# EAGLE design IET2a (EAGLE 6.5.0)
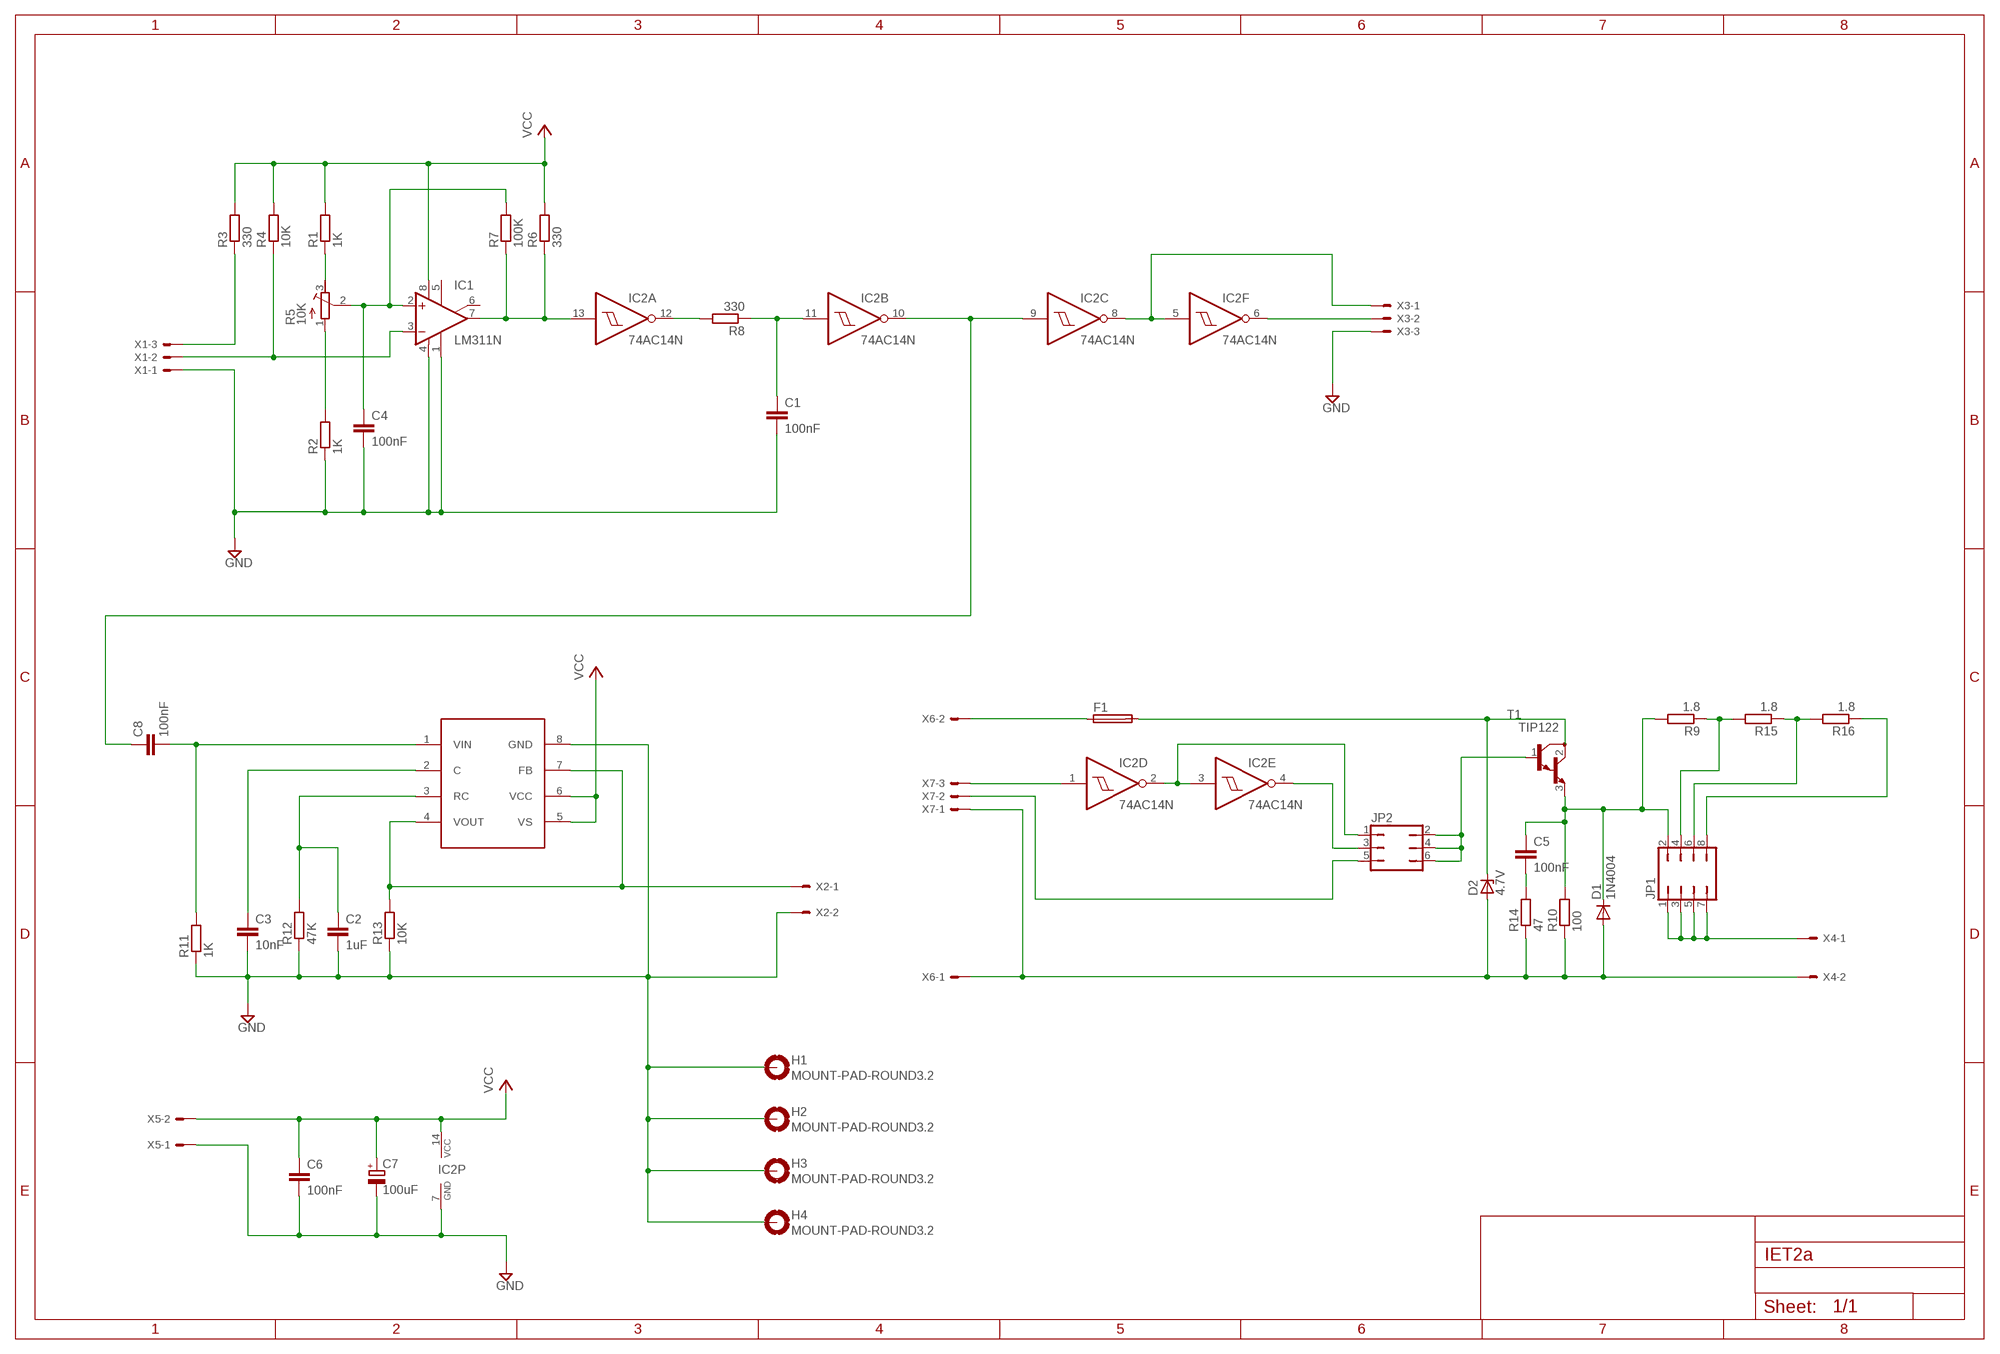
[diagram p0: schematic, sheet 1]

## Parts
C1  100nF  C-EU050-045X075  [C050-045X075]
C2  1uF  C-EU050-045X075  [C050-045X075]
C3  10nF  C-EU050-045X075  [C050-045X075]
C4  100nF  C-EU050-045X075  [C050-045X075]
C5  100nF  C-EU050-045X075  [C050-045X075]
C6  100nF  C-EU050-045X075  [C050-045X075]
C7  100uF  CPOL-EUE10-22.5  [EB22,5D]
C8  100nF  C-EU050-045X075  [C050-045X075]
D1  1N4004  [DO41-10]
D2  4.7V  1N4728  [DO41Z10]
F1  TE5  [TE5]
H1  MOUNT-PAD-ROUND3.2  [3,2-PAD]
H2  MOUNT-PAD-ROUND3.2  [3,2-PAD]
H3  MOUNT-PAD-ROUND3.2  [3,2-PAD]
H4  MOUNT-PAD-ROUND3.2  [3,2-PAD]
IC1  LM311N  [DIL08]
IC2  74AC14N  [DIL14]
IC4  LM2917A  [DIL08]
JP1  JP4Q  [JP4Q]
JP2  JP3Q  [JP3Q]
R1  1K  R-EU_0613/15  [P0613/15]
R2  1K  R-EU_0613/15  [P0613/15]
R3  330  R-EU_0613/15  [P0613/15]
R4  10K  R-EU_0613/15  [P0613/15]
R5  10K  R-TRIMM3299W  [RTRIM3299W]
R6  330  R-EU_0613/15  [P0613/15]
R7  100K  R-EU_0613/15  [P0613/15]
R8  330  R-EU_0613/15  [P0613/15]
R9  1.8  R-EU_0613/15  [P0613/15]
R10  100  R-EU_VTA56  [VTA56]
R11  1K  R-EU_0613/15  [P0613/15]
R12  47K  R-EU_0613/15  [P0613/15]
R13  10K  R-EU_0613/15  [P0613/15]
R14  47  R-EU_VTA56  [VTA56]
R15  1.8  R-EU_0613/15  [P0613/15]
R16  1.8  R-EU_0613/15  [P0613/15]
T1  TIP122  [TO220]
X1  KK-156-3  [KK-156-3]
X2  KK-156-2  [KK-156-2]
X3  KK-156-3  [KK-156-3]
X4  KK-156-2  [KK-156-2]
X5  KK-156-2  [KK-156-2]
X6  KK-156-2  [KK-156-2]
X7  KK-156-3  [KK-156-3]

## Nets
GND: C1.2 C2.2 C3.2 C4.2 C6.2 C7.- H1.B3,2(MOUNT) H2.B3,2(MOUNT) H3.B3,2(MOUNT) H4.B3,2(MOUNT) IC1.1(GND) IC1.4(V-) IC2.7(P:GND) IC4.8(GND) R2.1 R11.1 R12.1 R13.1 X1.1 X2.2 X3.3 X5.1
N$1: IC1.7(OUT) IC2.13(A:I) R6.1 R7.1
N$2: IC2.2(D:O) IC2.3(E:I) JP2.1
N$3: R3.1 X1.3
N$4: C5.2 R14.2
N$5: C1.1 IC2.11(B:I) R8.1
N$6: IC2.12(A:O) R8.2
N$7: R1.1 R5.3(A)
N$8: C4.1 IC1.2(+IN) R5.2(S) R7.2
N$9: IC1.3(-IN) R4.1 X1.2
N$10: R2.2 R5.1(E)
N$11: F1.1 X6.2
N$12: D2.C F1.2 T1.2(C)
N$13: D1.A D2.A R10.1 R14.1 X4.2 X6.1 X7.1
N$14: C5.1 D1.C JP1.2 R9.2 R10.2 T1.3(E)
N$15: JP1.4 R9.1 R15.2
N$16: IC2.1(D:I) X7.3
N$17: C8.1 IC2.9(C:I) IC2.10(B:O)
N$18: C3.1 IC4.2(C)
N$19: JP2.2 JP2.4 JP2.6 T1.1(B)
N$20: IC2.4(E:O) JP2.3
N$21: JP2.5 X7.2
N$22: C2.1 IC4.3(RC) R12.2
N$23: C8.2 IC4.1(VIN) R11.2
N$24: JP1.6 R15.1 R16.2
N$25: IC4.4(VOUT) IC4.7(FB) R13.2 X2.1
N$26: JP1.8 R16.1
N$27: JP1.1 JP1.3 JP1.5 JP1.7 X4.1
N$28: IC2.5(F:I) IC2.8(C:O) X3.1
N$29: IC2.6(F:O) X3.2
VCC: C6.1 C7.+ IC1.8(V+) IC2.14(P:VCC) IC4.5(VS) IC4.6(VCC) R1.2 R3.2 R4.2 R6.2 X5.2
Unconnected: IC1.5(ON) IC1.6(ON/STR)

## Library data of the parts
C1-C6 C8 = resistor:C-EU: CAPACITOR, European symbol
C7 = resistor:CPOL-EU: POLARIZED CAPACITOR, European symbol
D1 = diode:1N4004: DIODE
D2 = diode:1N4728: Z DIODE
F1 = fuse:TE5: FUSE; OC_FARNELL: unknown; OC_NEWARK: unknown
H1-H4 = holes:MOUNT-PAD-ROUND: MOUNTING PAD, round
IC1 = linear:LM311: COMPARATOR
IC2 = 74xx-eu:74*14: Hex schmitt trigger INVERTER
IC4 = IET:LM2917A
JP1 = jumper:JP4Q: JUMPER
JP2 = jumper:JP3Q: JUMPER
R1-R4 R6-R9 R11-R13 R15 R16 = resistor:R-EU_: RESISTOR, European symbol
R5 = resistor:R-TRIMM: Trimm resistor
R10 R14 = rcl:R-EU_: RESISTOR, European symbol
T1 = transistor:TIP122: NPN BIPOLAR DARLINGTON TRANSISTOR
X1 X3 X7 = con-molex:KK-156-3: KK 156 HEADER Source: http://www.molex.com/pdm_docs/sd/026604100_sd.pdf; OC_FARNELL: unknown; OC_NEWARK: unknown
X2 X4-X6 = con-molex:KK-156-2: KK 156 HEADER; OC_FARNELL: unknown; OC_NEWARK: unknown

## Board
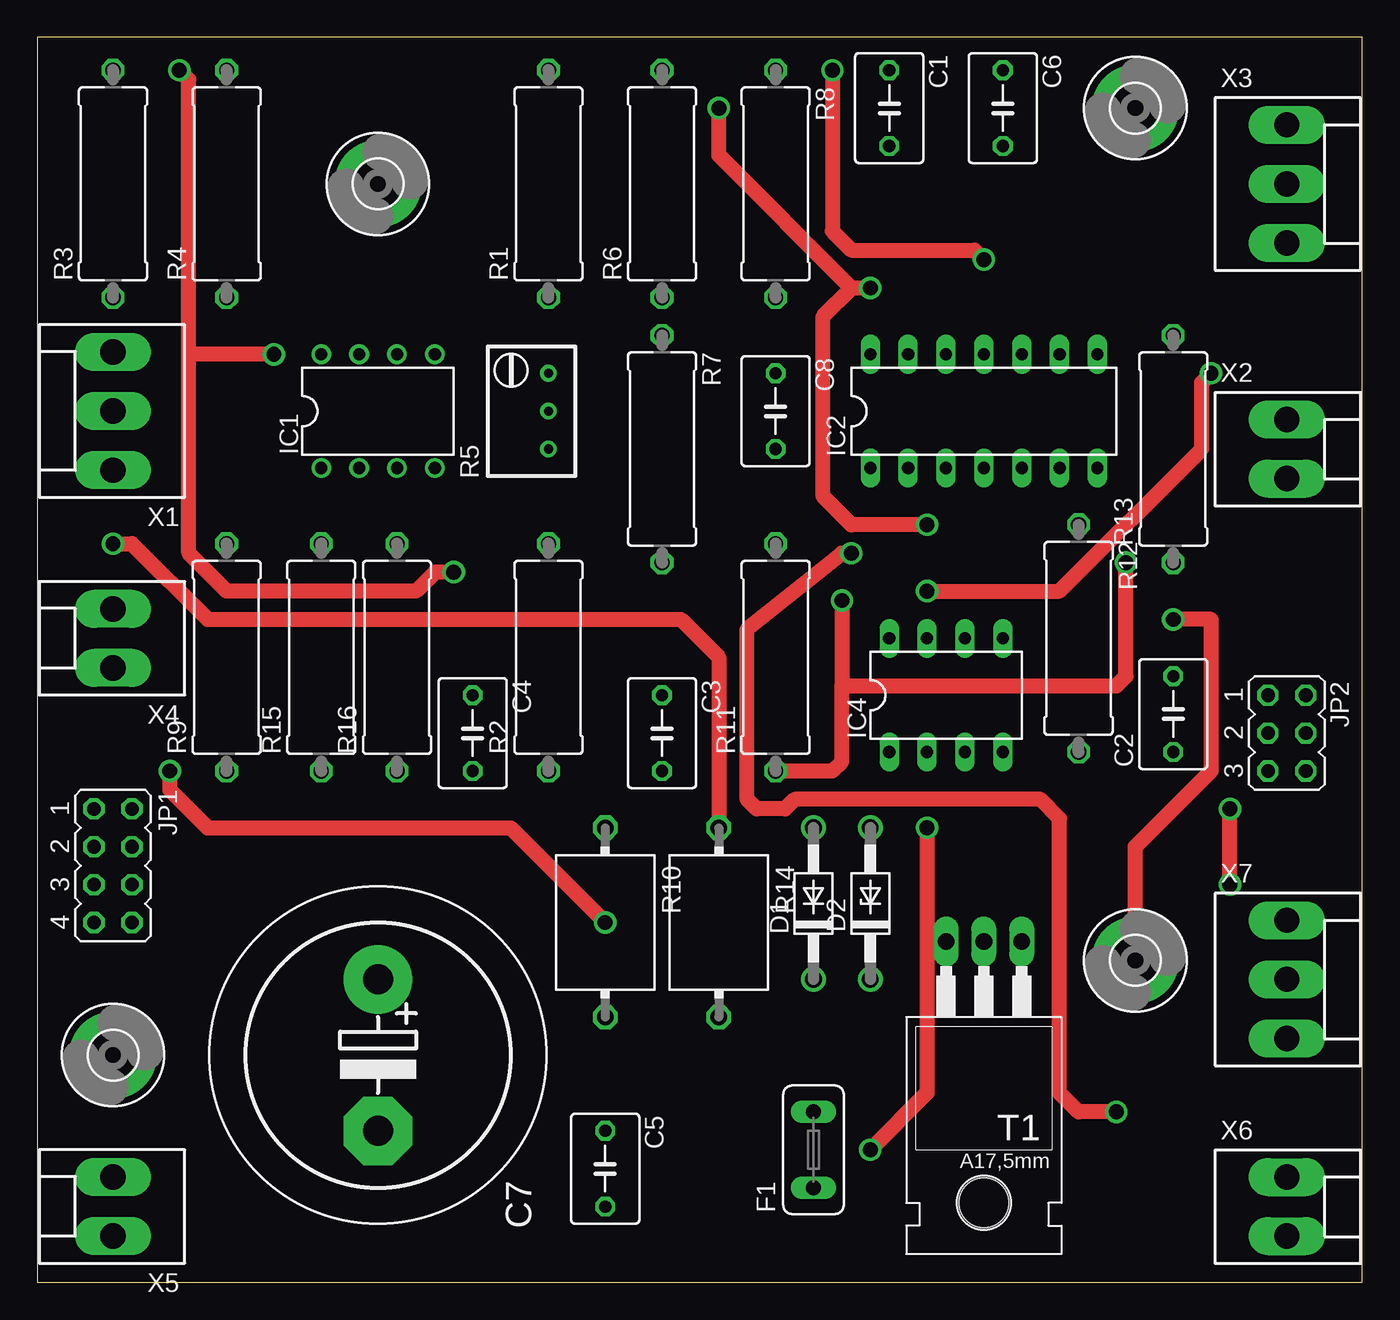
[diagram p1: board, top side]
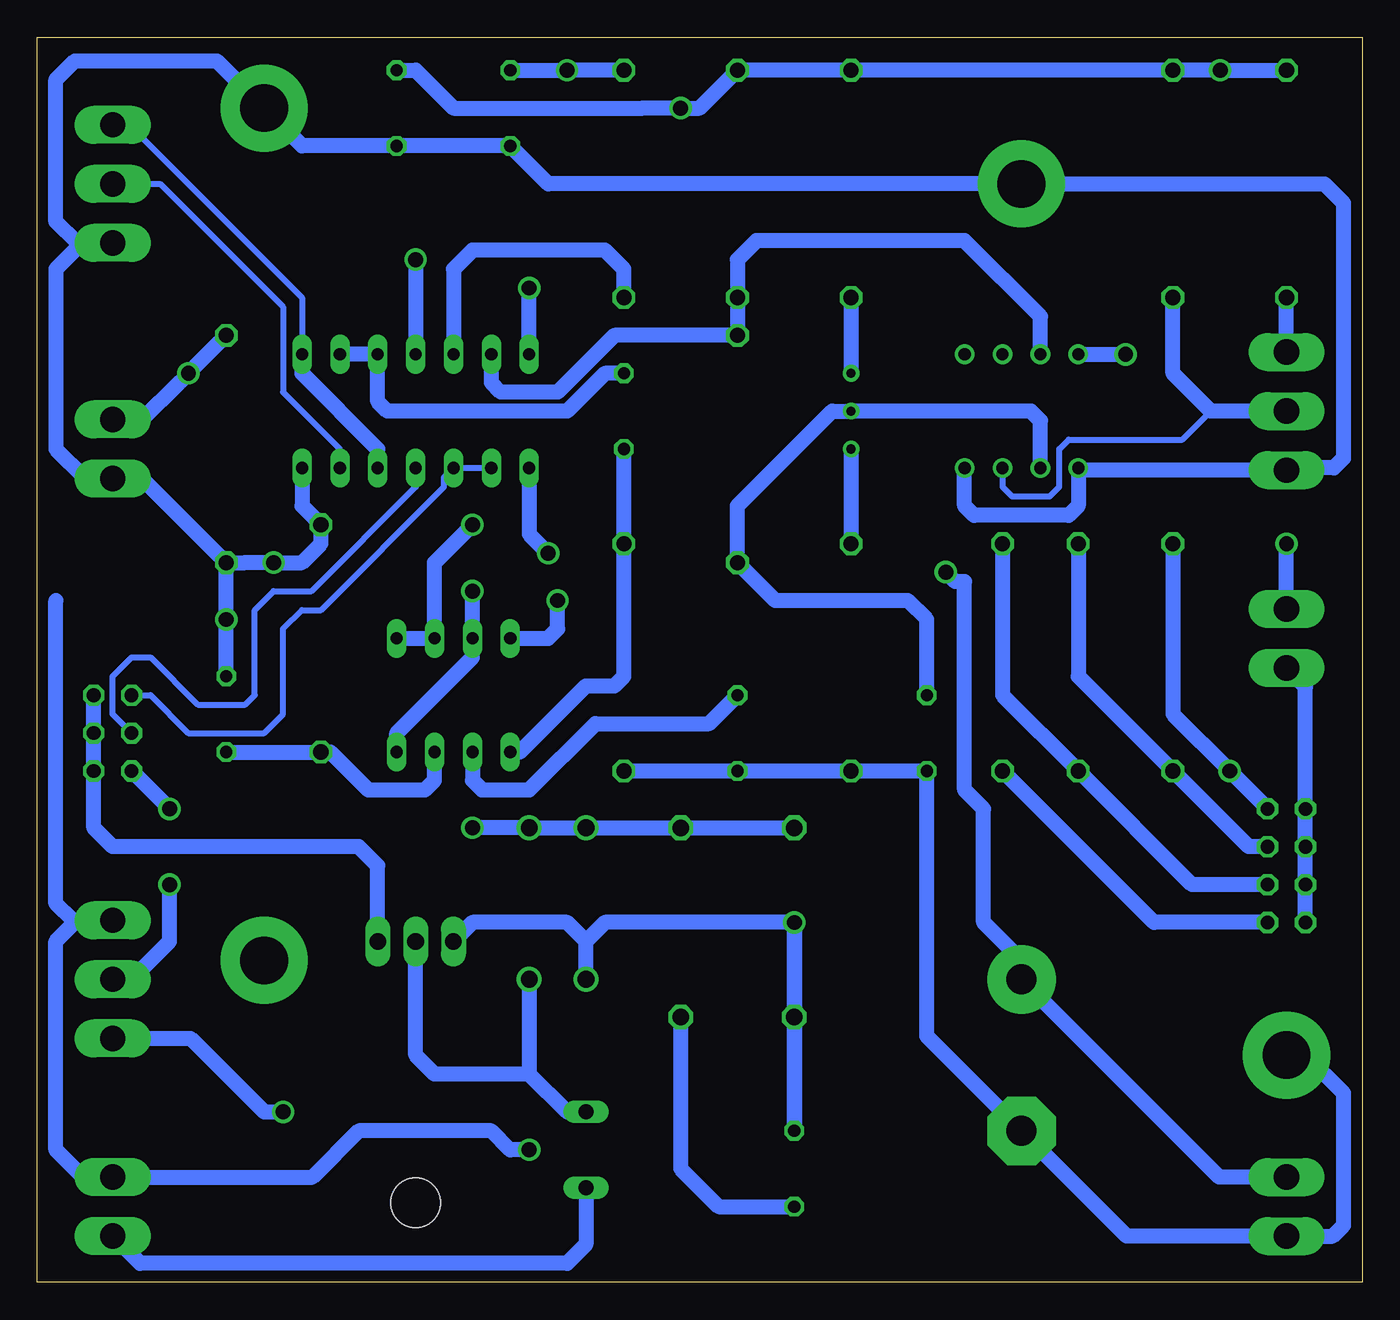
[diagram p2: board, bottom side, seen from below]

Size 88.88 x 83.49 mm. Coordinates in mm from the lower left corner, seen from the top.
Outline: 0,0 88.88,0 88.88,83.49 0,83.49 0,0
Copper layers (1*16): Top 0.035mm / dielectric 1.5mm / Bottom 0.035mm
Design rules "default": minimum track width 10mil, minimum drill 24mil, track to track 8mil, track to pad 8mil, pad to pad 8mil, via to via 8mil, smd to smd 8mil, copper to edge 40mil, drill to drill 8mil, minimum pad ring 10mil, minimum via ring 8mil, stop-mask expansion 4mil, vias tented up to drill 0mil, thermal gap 10mil

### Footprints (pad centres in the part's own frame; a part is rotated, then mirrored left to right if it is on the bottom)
C050-045X075 = drill 0.813 octagon: 1 -2.54,0; 2 2.54,0
EB22,5D = drill 2.007 pad 4.597: + -5.08,0 | drill 2.007 pad 4.597 octagon: - 5.08,0
DO41-10 = drill 1.118: A 5.08,0; C -5.08,0
DO41Z10 = drill 1.118: A 5.08,0; C -5.08,0
TE5 = drill 1.016 long: 1 -2.54,0; 2 2.54,0
3,2-PAD = drill 3.2 pad 5.842: B3,2 0,0
DIL08 = drill 0.813 pad 1.27: 1 -3.81,-3.81; 2 -1.27,-3.81; 3 1.27,-3.81; 4 3.81,-3.81; 5 3.81,3.81; 6 1.27,3.81; 7 -1.27,3.81; 8 -3.81,3.81
DIL14 = drill 0.813 long: 1 -7.62,-3.81; 2 -5.08,-3.81; 3 -2.54,-3.81; 4 0,-3.81; 5 2.54,-3.81; 6 5.08,-3.81; 7 7.62,-3.81; 8 7.62,3.81; 9 5.08,3.81; 10 2.54,3.81; 11 0,3.81; 12 -2.54,3.81; 13 -5.08,3.81; 14 -7.62,3.81
DIL08' = drill 0.813 long: 1 -3.81,-3.81; 2 -1.27,-3.81; 3 1.27,-3.81; 4 3.81,-3.81; 5 3.81,3.81; 6 1.27,3.81; 7 -1.27,3.81; 8 -3.81,3.81
JP4Q = drill 0.914 octagon: 1 -3.81,-1.27; 2 -3.81,1.27; 3 -1.27,-1.27; 4 -1.27,1.27; 5 1.27,-1.27; 6 1.27,1.27; 7 3.81,-1.27; 8 3.81,1.27
JP3Q = drill 0.914 octagon: 1 -2.54,-1.27; 2 -2.54,1.27; 3 0,-1.27; 4 0,1.27; 5 2.54,-1.27; 6 2.54,1.27
P0613/15 = drill 1.016 octagon: 1 -7.62,0; 2 7.62,0
RTRIM3299W = drill 0.61: 1 1.27,-2.54; 2 1.27,0; 3 1.27,2.54
VTA56 = drill 1.1 octagon: 1 -6.35,0; 2 6.35,0
TO220 = drill 1.118 long: 1 -2.54,-6.35; 2 0,-6.35; 3 2.54,-6.35 | hole 3.302: 0,11.176
KK-156-3 = drill 1.7 pad 2.184 long: 1 -3.96,0; 2 0,0; 3 3.96,0
KK-156-2 = drill 1.7 pad 2.184 long: 1 -1.98,0; 2 1.98,0

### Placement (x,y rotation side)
C1  57.15,78.74 270 top
C2  76.2,38.1 90 top
C3  41.91,36.83 270 top
C4  29.21,36.83 270 top
C5  38.1,7.62 270 top
C6  64.77,78.74 270 top
C7  22.86,15.24 270 top
C8  49.53,58.42 270 top
D1  52.07,25.4 90 top
D2  55.88,25.4 90 top
F1  52.07,8.89 90 top
H1  5.08,15.24 0 top
H2  22.86,73.66 0 top
H3  73.66,78.74 0 top
H4  73.66,21.59 0 top
IC1  22.86,58.42 0 top
IC2  63.5,58.42 0 top
IC4  LM2917A  [DIL08']  60.96,39.37 0 top
JP1  5.08,27.94 270 top
JP2  83.82,36.83 270 top
R1  34.29,73.66 90 top
R2  34.29,41.91 90 top
R3  5.08,73.66 90 top
R4  12.7,73.66 90 top
R5  33.02,58.42 0 top
R6  41.91,73.66 90 top
R7  41.91,55.88 270 top
R8  49.53,73.66 270 top
R9  12.7,41.91 90 top
R10  38.1,24.13 270 top
R11  49.53,41.91 90 top
R12  69.85,43.18 270 top
R13  76.2,55.88 90 top
R14  45.72,24.13 270 top
R15  19.05,41.91 90 top
R16  24.13,41.91 90 top
T1  63.5,16.51 180 top
X1  5.08,58.42 90 top
X2  83.82,55.88 270 top
X3  83.82,73.66 270 top
X4  5.08,43.18 90 top
X5  5.08,5.08 90 top
X6  83.82,5.08 270 top
X7  83.82,20.32 270 top

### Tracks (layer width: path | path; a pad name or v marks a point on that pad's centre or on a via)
GND  (via drill 1 pad 1.27)
  Top 1.016: H4.B3,2 73.66,29.21 78.74,34.29 78.74,44.45 v76.2,44.45 | R11.1 53.34,34.29 53.98,34.92 53.98,40.01 | v53.98,45.72 53.98,40.01 | 53.98,40.01 72.39,40.01 73.03,40.64 v73.03,48.26
  Bottom 1.016: X1.1 5.71,54.46 | 5.71,54.46 18.9,54.46 IC1.1 19.05,52.07 19.68,51.44 26.04,51.44 26.67,52.07 IC1.4 | R13.1 81.84,53.9 X2.2 83.89,53.98 85.72,53.98 87.63,55.88 87.63,67.94 85.88,69.7 X3.3 86.21,69.7 87.63,71.12 87.63,80.64 86.36,81.92 76.83,81.92 H3.B3,2 71.12,76.2 C6.2 C1.2 54.61,73.66 H2.B3,2 2.54,73.66 1.27,72.39 1.27,55.24 1.91,54.61 5.57,54.61 5.71,54.46 | R13.1 74.93,48.26 v73.03,48.26 71.12,48.26 69.85,49.53 R12.1 71.12,52.07 IC2.7 | C2.2 v76.2,44.45 R13.1 | R11.1 C3.2 R2.1 C4.2 29.21,16.51 C7.- 15.8,3.1 X5.1 1.98,3.1 1.27,3.81 1.27,12.7 3.81,15.24 H1.B3,2 | IC4.8 54.61,43.18 53.98,43.81 v53.98,45.72
N$1
  Bottom 1.016: IC1.7 21.59,64.77 26.67,69.85 40.64,69.85 41.91,68.58 R6.1 R7.1 50.16,63.5 53.98,59.69 57.78,59.69 58.42,60.33 IC2.13
N$2
  Bottom 0.406: JP2.1 81.28,39.37 78.74,36.83 73.66,36.83 72.39,38.1 72.39,43.81 71.12,45.09 69.85,45.09 61.59,53.34 61.59,53.98 IC2.3 IC2.2
N$3
  Bottom 1.016: X1.3 R3.1
N$4
  Bottom 1.016: R14.2 45.72,7.62 43.18,5.08 C5.2
N$5  (via drill 1 pad 1.27)
  Top 1.016: v53.34,81.28 53.34,70.48 54.61,69.22 62.87,69.22 v63.5,68.58
  Bottom 1.016: R8.1 v53.34,81.28 C1.1 | v63.5,68.58 IC2.11
N$6
  Bottom 1.016: R8.2 49.53,67.94 50.8,69.22 59.69,69.22 60.96,67.94 IC2.12
N$7
  Bottom 1.016: R1.1 R5.3
N$8
  Bottom 1.016: C4.1 29.21,44.45 30.48,45.72 39.37,45.72 R7.2 41.91,52.07 35.56,58.42 R5.2 22.23,58.42 21.59,57.78 IC1.2
N$9
  Bottom 0.406: IC1.3 24.13,53.34 23.5,52.7 20.95,52.7 20.32,53.34 20.32,55.88 19.68,56.52 12.06,56.52 10.16,58.42
  Bottom 1.016: X1.2 10.16,58.42 12.7,60.96 R4.1
N$10
  Bottom 1.016: R5.1 R2.2
N$11
  Bottom 1.016: F1.1 52.07,2.54 53.34,1.27 81.99,1.27 X6.2
N$12
  Bottom 1.016: F1.2 53.34,11.43 55.88,13.97 | 55.88,13.97 62.23,13.97 63.5,15.24 T1.2 | D2.C 55.88,13.97
N$13  (via drill 1 pad 1.27)
  Top 1.016: v5.08,49.53 6.35,49.53 11.43,44.45 43.18,44.45 45.72,41.91 R14.1 | v59.69,30.48 59.69,12.7 v55.88,8.89
  Bottom 1.016: R10.1 R14.1 D1.A D2.A v59.69,30.48 | X4.2 v5.08,49.53 | 87.63,45.72 87.63,25.4 86.51,24.28 X7.1 83.97,24.13 86.36,24.13 87.63,22.86 87.63,8.89 85.8,7.06 X6.1 70.41,7.06 67.31,10.16 58.42,10.16 57.15,8.89 v55.88,8.89
N$14  (via drill 1 pad 1.27)
  Top 1.016: v8.89,34.29 8.89,33.02 11.43,30.48 31.75,30.48 v38.1,24.13
  Bottom 1.016: JP1.2 v8.89,34.29 12.7,38.1 R9.2 | v38.1,24.13 R10.2 C5.1 v38.1,24.13 | D1.C 52.07,22.86 | 52.07,22.86 53.34,24.13 59.69,24.13 T1.3 | v38.1,24.13 50.8,24.13 52.07,22.86
N$15
  Bottom 1.016: JP1.4 7.62,29.21 R9.1 19.05,40.64 R15.2
N$16  (via drill 1 pad 1.27)
  Top 1.016: v72.39,11.43 69.85,11.43 68.58,12.7 68.58,31.11 67.31,32.38 50.8,32.38 50.16,31.75 48.26,31.75 47.62,32.38 47.62,43.81 53.98,48.9 v54.61,48.9
  Bottom 1.016: X7.3 78.59,16.36 73.66,11.43 v72.39,11.43 | IC2.1 55.88,50.16 v54.61,48.9
N$17
  Bottom 1.016: C8.1 50.8,60.96 53.34,58.42 65.41,58.42 66.04,59.05 IC2.10 IC2.9
N$18
  Bottom 1.016: IC4.2 59.69,33.66 59.05,33.02 55.88,33.02 51.44,37.47 43.81,37.47 C3.1
N$19
  Bottom 1.016: T1.1 66.04,27.94 67.31,29.21 83.82,29.21 85.09,30.48 JP2.6 JP2.4 JP2.2
N$20
  Bottom 0.406: JP2.3 83.82,38.1 83.82,40.64 82.55,41.91 81.28,41.91 78.11,38.73 74.93,38.73 74.3,39.37 74.3,45.09 73.03,46.35 70.48,46.35 63.5,53.34 IC2.4
N$21  (via drill 1 pad 1.27)
  Top 1.016: v80.01,26.67 v80.01,31.75
  Bottom 1.016: X7.2 82.55,20.32 80.01,22.86 v80.01,26.67 | v80.01,31.75 JP2.5
N$22
  Bottom 1.016: C2.1 R12.2 69.22,35.56 66.67,33.02 62.87,33.02 62.23,33.66 IC4.3
N$23
  Bottom 1.016: IC4.1 56.52,35.56 52.07,40.01 50.16,40.01 49.53,40.64 R11.2 C8.2
N$24
  Bottom 1.016: JP1.6 11.43,26.67 R15.1 24.13,39.37 R16.2
N$25  (via drill 1 pad 1.27)
  Top 1.016: v59.69,46.35 68.58,46.35 78.11,55.88 78.11,60.33 v78.74,60.96
  Bottom 1.016: X2.1 81.84,57.86 79.38,60.33 v78.74,60.96 R13.2 | IC4.4 64.77,36.83 59.69,41.91 IC4.7 v59.69,46.35
N$26
  Bottom 1.016: JP1.8 13.97,24.13 R16.1
N$27
  Bottom 1.016: JP1.7 JP1.5 JP1.3 JP1.1 3.81,39.93 X4.1
N$28
  Bottom 0.406: X3.1 82.7,77.62 71.12,66.04 IC2.8
  Bottom 1.016: IC2.5 66.04,55.88 71.12,60.96 IC2.8
N$29
  Bottom 0.406: X3.2 80.64,73.66 72.39,65.41 72.39,59.69 68.58,55.88 IC2.6
VCC  (via drill 1 pad 1.27)
  Top 1.016: v27.94,47.62 26.67,47.62 25.4,46.35 12.7,46.35 10.16,48.9 10.16,62.23 | 10.16,62.23 10.16,80.64 v9.53,81.28 | v15.88,62.23 10.16,62.23 | v59.69,50.8 54.61,50.8 52.7,52.7 52.7,64.77 54.61,66.67 | v55.88,66.67 54.61,66.67 | 54.61,66.67 45.72,75.56 v45.72,78.74
  Bottom 1.016: C6.1 63.5,81.28 60.96,78.74 48.26,78.74 v45.72,78.74 44.45,78.74 R6.2 R1.2 R4.2 v9.53,81.28 R3.2 | X5.2 9.6,7.06 C7.+ 22.86,21.59 25.4,24.13 25.4,31.75 26.67,33.02 26.67,46.99 27.3,46.99 v27.94,47.62 | IC4.5 IC4.6 62.23,48.26 v59.69,50.8 | IC1.8 v15.88,62.23 | IC2.14 v55.88,66.67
